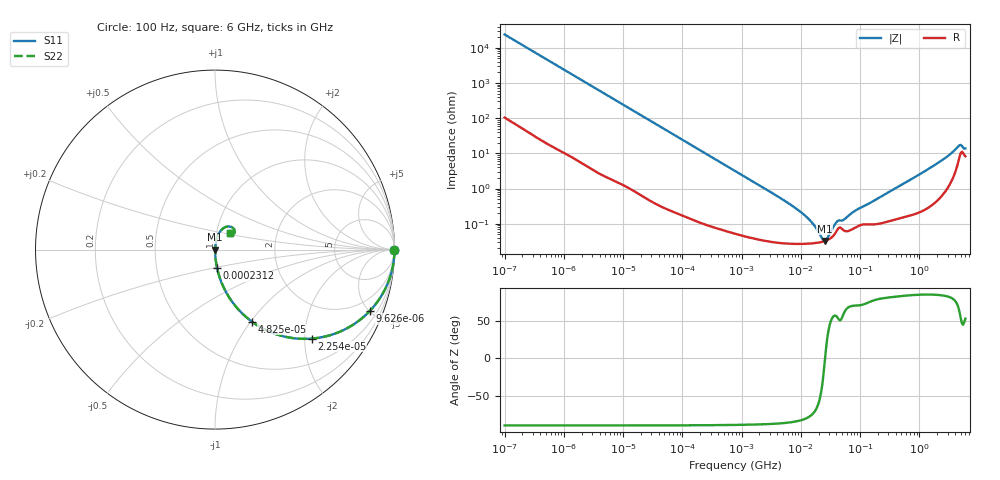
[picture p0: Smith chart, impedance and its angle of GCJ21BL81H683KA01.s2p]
!Murata Part Number: GCJ21BL81H683KA01
!These Parameters are Measured in Series Mode Connection
!Data Generated on Mar 13, 2026
!  o--ll--o
!Port1  Port2
!  o------o
!Operation Temp=25[degC], DC Bias Voltage=0[V]
!Freq. Start=100[Hz] Stop=6[GHz] 401[Steps]
# Hz S RI R 50
!Freq.(Hz) S11(Real) S11(Imag) S21(Real) S21(Imag) S12(Real) S12(Imag) S22(Real) S22(Imag)
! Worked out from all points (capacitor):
!   401 points, 100 Hz to 6 GHz, reference 50 ohm
!   read as one part in series: C = 66.3 nF near 109 Hz
!   lowest |Z| = 32.2 mohm at 25.46 MHz (marker M1)
!   series resonance near 25.67 MHz, so ESL is about 580 pH
!   S11 on the Smith chart (normalised r, x): 100 Hz: open; 9.626 kHz: 1.03, -5.04; 22.54 kHz: 1.01, -2.16; 48.25 kHz: 1.01, -1.01; 231.2 kHz: 1.00, -0.21; 6 GHz: 1.17, +0.22
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100  1 -0.00417  3.56e-05 0.00417  3.56e-05 0.00417  1 -0.00417
2008  0.9928 -0.0825  0.00722 0.0825  0.00722 0.0825  0.9928 -0.0825
5143  0.956 -0.2029  0.044 0.2029  0.044 0.2029  0.956 -0.2029
9626  0.8626 -0.3417  0.1374 0.3417  0.1374 0.3417  0.8626 -0.3417
22537  0.538 -0.4959  0.462 0.4959  0.462 0.4959  0.538 -0.4959
40335  0.2685 -0.4405  0.7315 0.4405  0.7315 0.4405  0.2685 -0.4405
48246  0.2047 -0.4007  0.7953 0.4007  0.7953 0.4007  0.2047 -0.4007
90302  0.0696 -0.2512  0.9304 0.2512  0.9304 0.2512  0.0696 -0.2512
231233  0.0121 -0.1046  0.9879 0.1046  0.9879 0.1046  0.0121 -0.1046
774597  0.00153 -0.0318  0.9985 0.0318  0.9985 0.0318  0.00153 -0.0318
6644369  0.000281 -0.00351  0.9997 0.00351  0.9997 0.00351  0.000281 -0.00351
1.555665e7  0.000277 -0.00102  0.9997 0.00102  0.9997 0.00102  0.000277 -0.00102
2.327686e7  0.000308 -0.000195  0.9997 0.000195  0.9997 0.000195  0.000308 -0.000195
2.545746e7  0.000321 -1.61e-05  0.9997 1.61e-05  0.9997 1.61e-05  0.000321 -1.61e-05
2.784235e7  0.00034 0.000165  0.9997 -0.000165  0.9997 -0.000165  0.00034 0.000165
4.165952e7  0.000687 0.000967  0.9993 -0.000967  0.9993 -0.000967  0.000687 0.000967
5.211241e7  0.00066 0.00108  0.9993 -0.00108  0.9993 -0.00108  0.00066 0.00108
8.527865e7  0.000803 0.00228  0.9992 -0.00228  0.9992 -0.00228  0.000803 0.00228
3.124326e8  0.00124 0.00799  0.9988 -0.00799  0.9988 -0.00799  0.00124 0.00799
1.95892e9  0.0068 0.0497  0.9932 -0.0497  0.9932 -0.0497  0.0068 0.0497
4.586474e9  0.0753 0.1294  0.9247 -0.1294  0.9247 -0.1294  0.0753 0.1294
6e9  0.0858 0.0932  0.9142 -0.0932  0.9142 -0.0932  0.0858 0.0932
